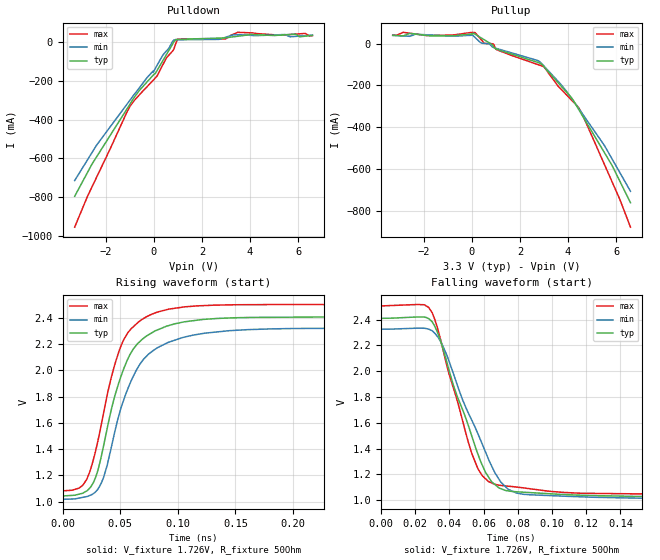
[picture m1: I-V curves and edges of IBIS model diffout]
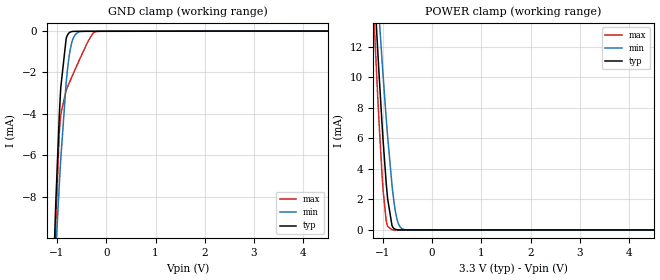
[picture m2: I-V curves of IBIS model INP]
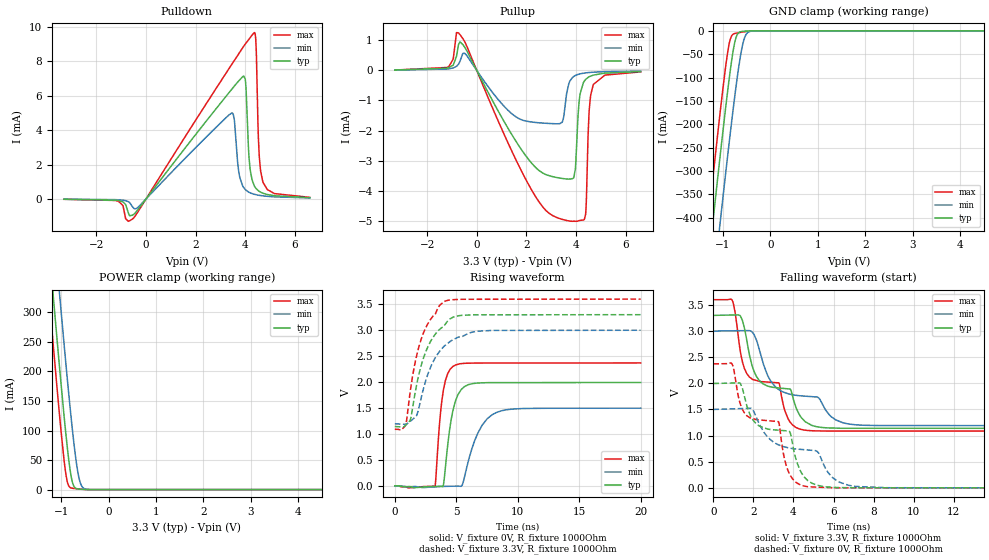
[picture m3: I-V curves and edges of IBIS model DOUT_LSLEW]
|Texas Instruments Incorporated
|LMX2572 6.4-GHz Low Power Wideband RF Synthesizer With Phase Synchronization
|and JESD204B Support
[IBIS Ver]   4.1
[File name]   lmx2572.ibs
[Date]   04/25/2018
[File Rev]   1.0
[Source]
| Texas Instruments Incorporated.
| Analog-eLab Design Center, HPA
| 12500 TI Blvd
| Dallas, TX -75243
[Notes]   Revision History:
| Rev 1.0: 04/25/2018
| - Initial version of the model
| - Model generated from simulations in SPECTRE
| - Warnings regarding combined Non-monotonicity of various models
|   have been reviewed and considered minor and can be ignored.
| - C_comp although listed in numerical order of value are
|   obtained from varying PVT conditions. For PVT conditions for
|   each specific value refer the buffer description under
|   respective [Model]. IBIS model user is responsible for using
|   appropriate C_comp to simulate for Signal Integrity.
[Disclaimer]
| This model is designed as an aid for customers of Texas Instruments.
| TI and its licensors and suppliers make no warranties, either expressed
| or implied, with respect to this  model, including the warranties of
| merchantability or fitness for a particular purpose. The model is
| provided solely on an "as is" basis. The entire risk as to its quality
| and performance is with the customer.
| This model is subject to change without notice. Texas Instruments
| Incorporated is not responsible for updating this model.
[Copyright]
(C) Copyright 2018 Texas Instruments Incorporated.All rights reserved.
|  Component LMX2572RHAR 40-pin VQFN - RHA package
|  Part # LMX2572RHAR
[Component]   LMX2572RHAR
[Manufacturer]  TI
[Package]   |40 VQFN- RHA package
|   typ   min   max
R_pkg   0.05   0.04   0.06
L_pkg   1.0nH   0.8nH   1.2nH
C_pkg   0.2pF   0.16pF   0.24pF
[Pin]  signal_name model_name R_pin L_pin C_pin
1   CE   nc   NA   NA   NA
2   GND   gnd   NA   NA   NA
3   VbiasVCO   nc   NA   NA   NA
4   GND   gnd   NA   NA   NA
5   SYNC   nc   NA   NA   NA
6   GND   gnd   NA   NA   NA
7   VccDIG   power   NA   NA   NA
8   OSCinP   nc   NA   NA   NA
9   OSCinM   nc   NA   NA   NA
10  VregIN   nc   NA   NA   NA
11  VccCP   power   NA   NA   NA
12  CPout   nc   NA   NA   NA
13  GND   gnd   NA   NA   NA
14  GND   gnd   NA   NA   NA
15  VccMASH   power   NA   NA   NA
16  SCK   INP   NA   NA   NA
17  SDI   INP   NA   NA   NA
18  RFoutBM   diffout   NA   NA   NA
19  RFoutBP   diffout   NA   NA   NA
20  MUXout   DOUT   NA   NA   NA
21  VccBUF   power   NA   NA   NA
22  RFoutAM   diffout   NA   NA   NA
23  RFoutAP   diffout   NA   NA   NA
24  CSB   INP   NA   NA   NA
25  GND   gnd   NA   NA   NA
26  VccVCO2   power   NA   NA   NA
27  VbiasVCO2   nc   NA   NA   NA
28  SysRefReq   nc   NA   NA   NA
29  VrefVCO2   nc   NA   NA   NA
30  RampClk   nc   NA   NA   NA
31  GND   gnd   NA   NA   NA
32  RampDir   nc   NA   NA   NA
33  VbiasVARAC   nc   NA   NA   NA
34  GND   gnd   NA   NA   NA
35  Vtune   nc   NA   NA   NA
36  VrefVCO   nc   NA   NA   NA
37  VccVCO   power   NA   NA   NA
38  VregVCO   nc   NA   NA   NA
39  GND   gnd   NA   NA   NA
40  GND   gnd   NA   NA   NA
[Diff pin]  inv_pin  vdiff  tdelay_typ  tdelay_min  tdelay_max
19   18   NA   0.0s   0.0s   0.0s
23   22   NA   0.0s   0.0s   0.0s
|   Model Selectors
[Model Selector] DOUT
DOUT_LSLEW   3.3V OUTPUT, low slew rate
DOUT_HSLEW   3.3V OUTPUT, high slew rate
| Models and submodels in the file (4): diffout (Output), INP (Input), DOUT_LSLEW (3-state), DOUT_HSLEW (3-state)
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|   diffout Model
[Model]   diffout
Model_type   Output
Polarity   Non-Inverting
Vmeas = 1.726
Vref = 1.726
Cref = 2pF
Rref = 50
|   typ   min   max
|   (nom PVT)   (fast PVT)   (slow PVT)
C_comp   1.674E-13   1.598E-13   1.835E-13
| Where nom  PVT is Nominal Process, 3.3V, 27C
|   Fast PVT is Strong Process,  3.45V, -40C
|   Slow PVT is Weak Process,   3.15V, 105C
[Voltage Range]   3.3   3.15   3.45
|Junction Temperature
[Temperature Range]   27   105   -40
[Pullup Reference]   3.3   3.15   3.45
[Pulldown Reference]   -0   -0   0
[Power Clamp Reference]   3.3   3.15   3.45
[GND Clamp Reference]   0   0   0
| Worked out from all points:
|   slope of the pulldown table from 0 to 0.495 V, typ, clamps not added: 5.13 ohm
|   slope of the pullup table from 0 to 0.495 V, typ, clamps not added: 18.9 ohm
|   falling waveform, V_fixture 1.726V, R_fixture 50Ohm: 20-80 % time 20.7ps typ, 24ps min, 17.7ps max; typ from 2.41 V to 1.04 V
|   rising waveform, V_fixture 1.726V, R_fixture 50Ohm: 20-80 % time 26.6ps typ, 29.7ps min, 24.2ps max; typ from 1.04 V to 2.41 V
[Pulldown]
|   Voltage   I(typ)   I(min)   I(max)
-3.3V     -795.7mA   -714.5mA   -954.6mA
-2.389V   -592.7mA   -532.4mA   -698.1mA
-1.094V   -340mA     -316.6mA   -354.4mA
-602.3mV  -249.5mA   -235.9mA   -272.5mA
121mV     -149.6mA   -122.9mA   -177.3mA
511.5mV   -67.39mA   -48.1mA    -84.35mA
775.1mV   -11.91mA   2.074mA    -46.99mA
993.4mV   13.12mA    10.84mA    13.58mA
2.952V    20.56mA    22.38mA    15.38mA
3.492V    29.1mA     36.66mA    49.3mA
6.287V    29.33mA    31.93mA    43.62mA
6.6V      33.63mA    34.8mA     32.26mA
[Pullup]
|   Voltage   I(typ)   I(min)   I(max)
-3.3V     39mA       38.87mA    40.21mA
-33.65mV  44.86mA    44.68mA    52.87mA
121mV     44.93mA    29.71mA    52.29mA
511.5mV   17.82mA    196.6uA    1.165mA
889.7mV   -13.42mA   -18.05mA   -2.025mA
1.054V    -27.64mA   -24.7mA    -30.72mA
2.739V    -90.02mA   -81.33mA   -100.3mA
3.002V    -111.5mA   -108.1mA   -112.2mA
4.137V    -258.3mA   -259.6mA   -268.6mA
4.59V     -342.7mA   -334mA     -336.8mA
5.834V    -581.9mA   -550.7mA   -659.8mA
6.6V      -759.5mA   -704.9mA   -875.9mA
[Ramp]
R_load = 50
|   typ   min   max
dV/dt_r   0.818384/2.65739e-11   0.78342/2.96623e-11   0.851942/2.41976e-11
dV/dt_f   0.820126/2.06866e-11   0.784654/2.40153e-11   0.854303/1.76748e-11
[Falling Waveform]
V_fixture = 1.726V
V_fixture_min = 1.639V
V_fixture_max = 1.83V
R_fixture = 50Ohm
C_fixture = 0F
|   Time   V(typ)   V(min)   V(max)
0s        2.41V      2.325V     2.506V
25.42ps   2.419V     2.333V     2.515V
30ps      2.383V     2.313V     2.453V
35.52ps   2.208V     2.216V     2.212V
53.16ps   1.496V     1.619V     1.361V
59.35ps   1.269V     1.431V     1.188V
64.65ps   1.143V     1.267V     1.133V
74.35ps   1.072V     1.084V     1.108V
106.1ps   1.044V     1.031V     1.06V
2ns       1.043V     1.017V     1.082V
[Rising Waveform]
V_fixture = 1.726V
V_fixture_min = 1.639V
V_fixture_max = 1.83V
R_fixture = 50Ohm
C_fixture = 0F
|   Time   V(typ)   V(min)   V(max)
0s        1.043V     1.017V     1.082V
17.61ps   1.065V     1.033V     1.126V
26.48ps   1.143V     1.06V      1.317V
35.52ps   1.428V     1.186V     1.678V
44.03ps   1.766V     1.487V     2.008V
56.44ps   2.085V     1.858V     2.285V
74.35ps   2.27V      2.122V     2.415V
106.1ps   2.37V      2.254V     2.484V
275.2ps   2.406V     2.322V     2.501V
2ns       2.407V     2.323V     2.502V
|   Model INP
[Model]   INP
Model_type   Input
Vinl = .4
Vinh = 1.4
|   typ   min   max
|   (nom PVT)   (slow PVT)   (fast PVT)
C_comp   0.097p   0.055p   0.172p
| Where nom  PVT is Nominal Process, 3.3V, 27C
|   Fast PVT is Strong Process,  3.6V, -40C
|   Slow PVT is Weak Process,   3V, 125C
[Voltage Range]   3.3   3   3.6
|Junction Temperature
[Temperature Range]   27   125   -40
[Power Clamp Reference]   3.3   3   3.6
[GND Clamp Reference]   0   0   0
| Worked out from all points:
|   GND clamp passes 1 mA (typ) near -0.84 V on its own axis
|   POWER clamp passes 1 mA (typ) near -0.85 V on its own axis
[GND Clamp]
|   Voltage   I(typ)   I(min)   I(max)
-3.3V     -246.7mA   -151.3mA   -472.5mA
-1.063V   -10.99mA   -12.47mA   -13.38mA
-1.043V   -9.526mA   -11.49mA   -11.15mA
-1.033V   -8.823mA   -11.01mA   -10.14mA
-1.023V   -8.14mA    -10.54mA   -9.21mA
-953.7mV  -4.036mA   -7.394mA   -4.875mA
-924mV    -2.719mA   -6.164mA   -4.026mA
-815.1mV  -359.4uA   -2.508mA   -2.855mA
-726mV    -41.2uA    -819.4uA   -2.358mA
-597.3mV  -10.68uA   -94.98uA   -1.663mA
-211.2mV  -9.103uA   -7.806uA   -22.77uA
6.6V      0A         0A         0A
[POWER Clamp]
|   Voltage   I(typ)   I(min)   I(max)
-3.3V     164.1mA    142.7mA    184.6mA
-1.27V    21.95mA    24.01mA    20.35mA
-1.162V   15.17mA    18.29mA    12.57mA
-1.112V   12.23mA    15.77mA    9.255mA
-1.073V   9.96mA     13.8mA     6.765mA
-993.3mV  5.782mA    10.03mA    2.547mA
-924mV    2.765mA    6.978mA    472uA
-815.1mV  299.5uA    2.966mA    9.519uA
-755.7mV  53.96uA    1.431mA    2.479uA
-696.3mV  9.978uA    523.6uA    1.72uA
-537.9mV  1.219uA    16.89uA    1.015uA
6.6V      0A         0A         0A
|   Model DOUT_LSLEW
[Model]   DOUT_LSLEW
Model_type   3-state
Polarity   Non-Inverting
Vmeas = 1.65
Vref = 3.3
Cref = 1pF
Rref = 1000
|   typ   min   max
|   (nom PVT)   (fast PVT)   (slow PVT)
C_comp   1.019p   0.968p   1.051p
| Where nom  PVT is Nominal Process, 3.3V, 27C
|   Fast PVT is Strong Process,  3.6V, -40C
|   Slow PVT is Weak Process,   3V, 125C
[Voltage Range]   3.3   3   3.6
|Junction Temperature
[Temperature Range]   27   125   -40
[Pullup Reference]   3.3   3   3.6
[Pulldown Reference]   0   0   0
[Power Clamp Reference]   3.3   3   3.6
[GND Clamp Reference]   0   0   0
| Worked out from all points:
|   slope of the pulldown table from 0 to 0.495 V, typ, clamps not added: 528 ohm
|   slope of the pullup table from 0 to 0.495 V, typ, clamps not added: 627 ohm
|   GND clamp passes 1 mA (typ) near -0.57 V on its own axis
|   POWER clamp passes 1 mA (typ) near -0.63 V on its own axis
|   falling waveform, V_fixture 3.3V, R_fixture 1000Ohm: 20-80 % time 2.45ns typ, 3.22ns min, 2.31ns max; typ from 3.3 V to 1.14 V
|   rising waveform, V_fixture 0V, R_fixture 1000Ohm: 20-80 % time 749ps typ, 1.4ns min, 569ps max; typ from 0 V to 1.99 V
|   rising waveform, V_fixture 3.3V, R_fixture 1000Ohm: 20-80 % time 1.63ns typ, 1.79ns min, 1.49ns max; typ from 1.14 V to 3.3 V
|   falling waveform, V_fixture 0V, R_fixture 1000Ohm: 20-80 % time 2.61ns typ, 3.39ns min, 2.43ns max; typ from 2 V to 0 V
[Pulldown]
|   Voltage   I(typ)   I(min)   I(max)
-3.3V     -11.43uA   -7.802uA   -12.1uA
-537.9mV  -936.6uA   -451.7uA   -1.153mA
3.462V    6.382mA    4.997mA    7.828mA
3.759V    6.891mA    1.418mA    8.479mA
3.937V    7.142mA    671.1uA    8.867mA
4.016V    6.747mA    535.7uA    9.031mA
4.165V    2.21mA     385.6uA    9.304mA
4.372V    751.3uA    275.1uA    9.665mA
4.442V    605.9uA    250.9uA    8.713mA
4.561V    452.6uA    217.8uA    2.597mA
4.709V    342.4uA    186.9uA    1.005mA
6.6V      81.82uA    66.05uA    100.7uA
[GND Clamp]
|   Voltage   I(typ)   I(min)   I(max)
-3.3V     -2.452A    -2.589A    -2.364A
-1.439V   -627.2mA   -770.9mA   -533mA
-1.27V    -466.7mA   -610.7mA   -372.2mA
-1.211V   -410.7mA   -554.6mA   -316.2mA
-1.073V   -282mA     -425.3mA   -188.4mA
-1.033V   -246mA     -388.8mA   -153.2mA
-874.5mV  -109.2mA   -246.3mA   -31.62mA
-765.6mV  -33.07mA   -153.9mA   -6.398mA
-696.3mV  -7.92mA    -99.78mA   -4.642mA
-577.5mV  -1.073mA   -27.36mA   -2.516mA
-419.1mV  -88.15uA   -1.084mA   -769.1uA
6.6V      0A         0A         0A
[Pullup]
|   Voltage   I(typ)   I(min)   I(max)
-3.3V     12.07uA    9.347uA    12.51uA
-1.132V   89.8uA     52.94uA    125.7uA
-735.9mV  862.4uA    206.3uA    1.249mA
2.234V    -3.109mA   -1.72mA    -4.015mA
3.432V    -3.594mA   -1.729mA   -4.955mA
3.858V    -3.601mA   -234.1uA   -5.021mA
3.977V    -3.257mA   -167uA     -5.022mA
4.145V    -883.9uA   -117.5uA   -4.995mA
4.382V    -304.1uA   -82.23uA   -4.8mA
4.521V    -215.1uA   -69.84uA   -1.435mA
4.699V    -155.4uA   -58.43uA   -464.3uA
6.6V      -38.28uA   -21.08uA   -49.46uA
[POWER Clamp]
|   Voltage   I(typ)   I(min)   I(max)
-3.3V     2.408A     2.526A     2.331A
-1.389V   536.7mA    662mA      454.1mA
-1.231V   386.9mA    512.5mA    303.9mA
-1.171V   331.5mA    457.1mA    248.6mA
-1.053V   223.1mA    347.7mA    141.4mA
-1.013V   188mA      311.9mA    107.5mA
-894.3mV  88.96mA    207.3mA    22.7mA
-795.3mV  24.72mA    125.6mA    2.896mA
-735.9mV  6.329mA    81.34mA    1.968mA
-636.9mV  1.065mA    24.47mA    1.107mA
-478.5mV  181.4uA    709.5uA    176.1uA
6.6V      0A         0A         0A
[Ramp]
R_load = 1000
|   typ   min   max
dV/dt_r   1.19558/7.49454e-10   0.89825/1.40115e-09   1.4217/5.69081e-10
dV/dt_f   1.29663/2.44804e-09   1.08511/3.20365e-09   1.50804/2.31143e-09
[Falling Waveform]
V_fixture = 3.3V
V_fixture_min = 3V
V_fixture_max = 3.6V
R_fixture = 1000Ohm
C_fixture = 0F
|   Time   V(typ)   V(min)   V(max)
0s        3.3V       3V         3.6V
928.8ps   3.307V     3.005V     3.597V
1.34ns    3.295V     3.007V     2.629V
1.669ns   2.822V     3.008V     2.186V
2.149ns   2.133V     2.83V      2.054V
3.27ns    1.91V      1.88V      2.009V
3.726ns   1.894V     1.801V     1.326V
4.301ns   1.398V     1.763V     1.126V
7.116ns   1.14V      1.206V     1.087V
20ns      1.139V     1.191V     1.087V
[Rising Waveform]
V_fixture = 0V
V_fixture_min = 0V
V_fixture_max = 0V
R_fixture = 1000Ohm
C_fixture = 0F
|   Time   V(typ)   V(min)   V(max)
0s        108.1nV    2.108uV    192.6nV
3.27ns    -11.22mV   -20.47mV   -5.748mV
3.646ns   -8.576mV   -15.22mV   1.222V
3.959ns   25.78mV    -12.06mV   1.856V
4.475ns   1.109V     -8.854mV   2.236V
4.982ns   1.663V     -6.554mV   2.334V
5.506ns   1.879V     28.86mV    2.359V
7.116ns   1.986V     1.173V     2.367V
8.316ns   1.989V     1.42V      2.368V
20ns      1.993V     1.497V     2.369V
[Rising Waveform]
V_fixture = 3.3V
V_fixture_min = 3V
V_fixture_max = 3.6V
R_fixture = 1000Ohm
C_fixture = 0F
|   Time   V(typ)   V(min)   V(max)
0s        1.143V     1.197V     1.09V
895.1ps   1.171V     1.19V      1.179V
1.276ns   1.282V     1.246V     1.854V
1.754ns   1.92V      1.348V     2.487V
2.149ns   2.324V     1.699V     2.83V
2.7ns     2.688V     2.161V     3.13V
3.959ns   3.069V     2.678V     3.546V
4.913ns   3.265V     2.838V     3.592V
6.751ns   3.297V     2.982V     3.597V
20ns      3.3V       3V         3.6V
[Falling Waveform]
|Gnd
V_fixture = 0V
V_fixture_min = 0V
V_fixture_max = 0V
R_fixture = 1000Ohm
C_fixture = 0F
|   Time   V(typ)   V(min)   V(max)
0s        1.997V     1.5V       2.373V
928.8ps   2.005V     1.511V     2.376V
1.361ns   1.988V     1.517V     1.589V
1.669ns   1.573V     1.52V      1.381V
2.149ns   1.222V     1.348V     1.305V
3.248ns   1.103V     824mV      1.268V
3.726ns   1.089V     767mV      330.1mV
4.499ns   228.9mV    731.5mV    37.34mV
7.116ns   2.047mV    26.75mV    744.9uV
20ns      -35.77uV   -26.42uV   -32.15uV
